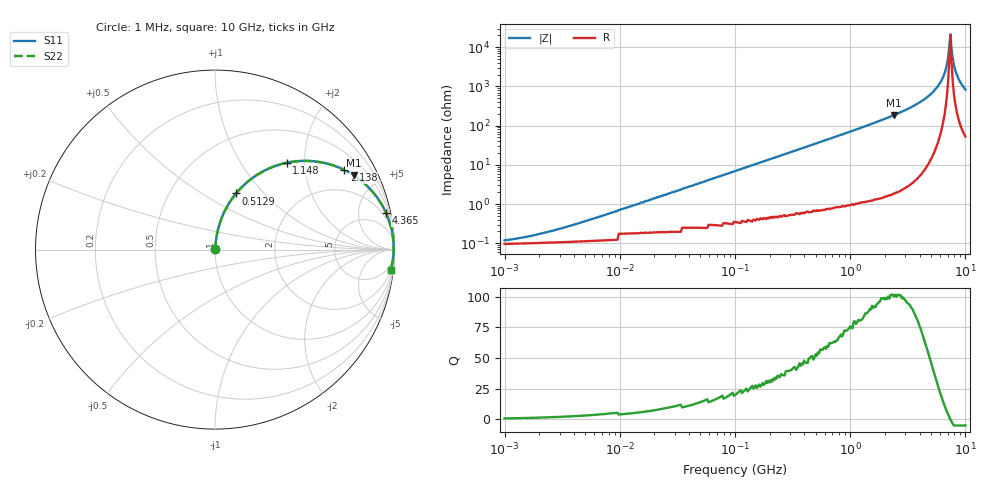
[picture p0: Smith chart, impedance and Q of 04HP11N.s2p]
# MHz S MA R 50
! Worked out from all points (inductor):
!   401 points, 1 MHz to 10 GHz, reference 50 ohm
!   read as one part in series: L = 11 nH near 4.898 MHz
!   highest Q = 101 at 2.399 GHz (marker M1), where L = 12.3 nH
!   self-resonance near 7.244 GHz
!   S11 on the Smith chart (normalised r, x): 1 MHz: 1.00, +0.00; 512.9 MHz: 1.01, +0.71; 1.148 GHz: 1.02, +1.63; 2.138 GHz: 1.03, +3.22; 4.365 GHz: 1.16, +9.24; 10 GHz: 2, -17
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1  0.001147 37.0  0.999 -0.0  0.999 -0.0  0.001147 37.0
4.677  0.003454 69.0  0.999 -0.2  0.999 -0.2  0.003454 69.0
21.878  0.015 82.0  0.998 -0.9  0.998 -0.9  0.015 82.0
102.329  0.07 83.3  0.994 -4.0  0.994 -4.0  0.07 83.3
467.735  0.307 71.0  0.946 -17.9  0.946 -17.9  0.307 71.0
512.861  0.334 69.4  0.936 -19.5  0.936 -19.5  0.334 69.4
1148.154  0.627 50.5  0.771 -38.8  0.771 -38.8  0.627 50.5
2137.962  0.846 31.7  0.525 -57.8  0.525 -57.8  0.846 31.7
2187.762  0.852 31.0  0.514 -58.5  0.514 -58.5  0.852 31.0
2398.833  0.876 28.2  0.473 -61.2  0.473 -61.2  0.876 28.2
4365.158  0.974 12.2  0.211 -77.0  0.211 -77.0  0.974 12.2
5370.318  0.989 7.3  0.126 -81.2  0.126 -81.2  0.989 7.3
6165.95  0.994 4.1  0.072 -82.9  0.072 -82.9  0.994 4.1
6606.934  0.995 2.5  0.045 -82.2  0.045 -82.2  0.995 2.5
6918.31  0.995 1.5  0.027 -79.3  0.027 -79.3  0.995 1.5
7079.458  0.995 1.0  0.018 -74.9  0.018 -74.9  0.995 1.0
7413.102  0.995 -0.0  0.004694 4.6  0.004694 4.6  0.995 -0.0
7585.776  0.995 -0.5  0.011 62.1  0.011 62.1  0.995 -0.5
8128.305  0.994 -2.1  0.037 79.5  0.037 79.5  0.994 -2.1
8511.38  0.993 -3.1  0.054 80.9  0.054 80.9  0.993 -3.1
9332.543  0.989 -5.2  0.09 80.6  0.09 80.6  0.989 -5.2
10000  0.986 -6.7  0.118 79.6  0.118 79.6  0.986 -6.7
